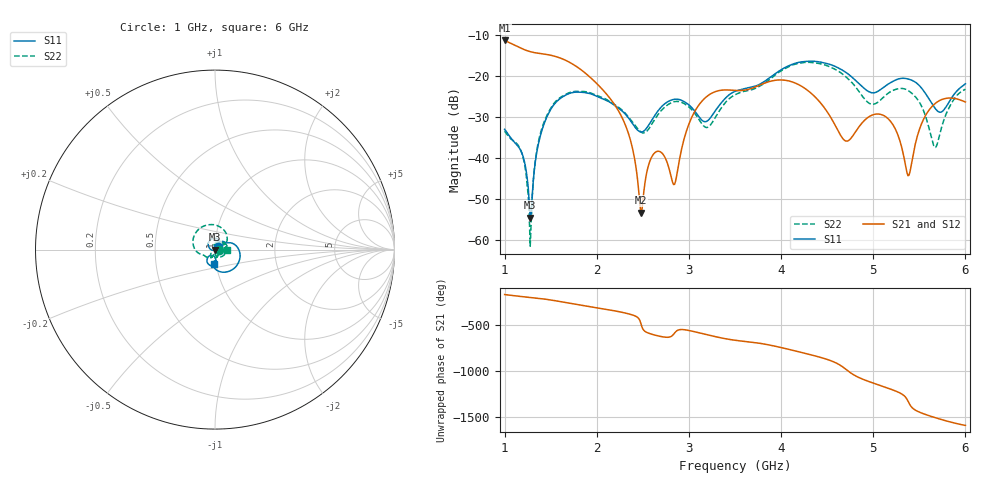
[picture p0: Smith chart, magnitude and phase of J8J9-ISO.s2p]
!Agilent Technologies,E8364B,MY43040528,A.07.50.67
!Agilent E8364B: A.07.50.67
!Date: Sunday, March 01, 2026 17:10:18
!Correction: S11(Full 2 Port(1,2))
!S21(Full 2 Port(1,2))
!S12(Full 2 Port(1,2))
!S22(Full 2 Port(1,2))
!S2P File: Measurements: S11, S21, S12, S22:
# Hz S  dB  R 50
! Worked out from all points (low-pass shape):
!   451 points, 1 GHz to 6 GHz, reference 50 ohm
!   highest |S21| = -11.40 dB at 1 GHz (marker M1); lowest = -53.4 dB at 2.478 GHz (marker M2)
!   |S21| within 3 dB of the highest: start of sweep to 1.332 GHz
!   lowest |S11| = -54.6 dB at 1.278 GHz (marker M3), VSWR 1.00, Z = 50.1 - j0.129 ohm
!   |S11| at or under -10 dB: start of sweep to end of sweep
!   |S22| runs from -61.6 to -16.7 dB; largest |S21 - S12| = 0.0013
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1e9  -33.07 40.7  -11.40 -167.5  -11.44 -167.4  -33.55 -2.9
1.188889e9  -38.97 32.1  -13.40 170.2  -13.44 170.2  -39.06 -8.9
1.277778e9  -54.61 -43.9  -14.13 161.4  -14.17 161.4  -61.60 39.7
1.355556e9  -37.89 -161.0  -14.49 153.2  -14.53 153.3  -37.41 120.9
1.444444e9  -30.82 170.2  -14.77 141.7  -14.81 141.7  -30.41 96.9
1.844444e9  -24.06 85.2  -18.81 74.2  -18.84 74.3  -23.84 -5.0
2.288889e9  -28.90 36.2  -30.90 -3.7  -30.93 -3.7  -28.69 -78.3
2.388889e9  -31.72 36.0  -37.84 -30.1  -37.88 -30.1  -31.34 -86.9
2.477778e9  -33.72 51.7  -53.39 -118.6  -53.48 -118.4  -33.73 -77.1
2.566667e9  -31.96 74.2  -41.48 131.0  -41.52 131.1  -32.90 -57.5
2.666667e9  -28.53 74.5  -38.43 102.5  -38.47 102.6  -29.42 -59.4
2.844444e9  -25.75 49.7  -46.51 134.1  -46.54 134.2  -26.33 -93.3
3.088889e9  -29.42 25.2  -27.77 141.8  -27.82 141.8  -29.97 -135.8
3.211111e9  -30.84 47.9  -24.78 112.1  -24.83 112.2  -32.50 -118.0
3.5e9  -23.83 45.1  -23.59 55.5  -23.63 55.6  -24.67 -128.4
4.344444e9  -16.46 -39.8  -24.65 -108.1  -24.69 -108.0  -16.80 111.4
4.7e9  -19.14 -88.0  -35.92 102.4  -35.96 102.4  -20.22 46.1
4.966667e9  -24.05 -91.6  -29.84 -38.5  -29.88 -38.5  -26.85 34.7
5.166667e9  -21.99 -83.2  -30.61 -108.0  -30.65 -108.0  -24.19 38.9
5.377778e9  -20.80 -109.6  -44.41 112.7  -44.45 112.7  -23.61 -2.3
5.666667e9  -27.81 -125.5  -26.88 -64.4  -26.93 -64.4  -37.50 -8.3
6e9  -21.99 -93.9  -26.42 -150.8  -26.46 -150.8  -23.29 -0.8
